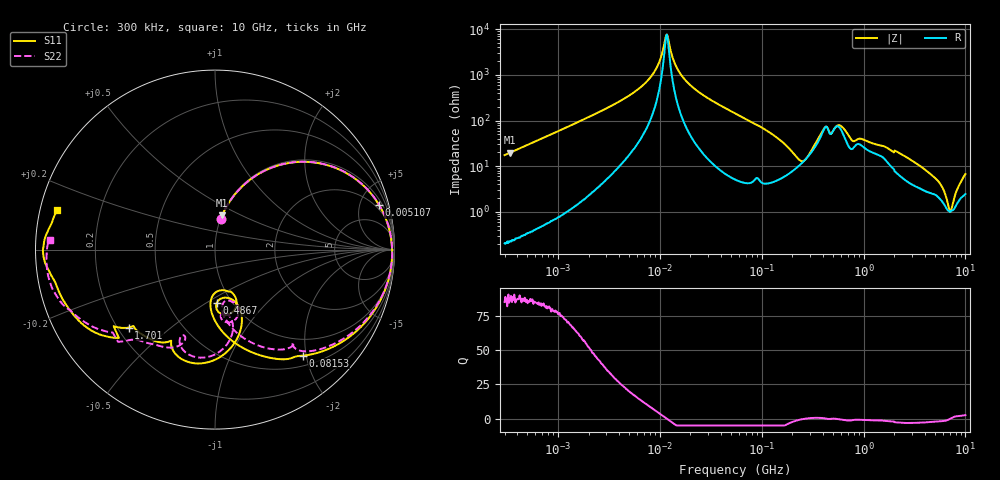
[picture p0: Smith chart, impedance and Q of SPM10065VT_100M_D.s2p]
! S-Parameter Data Generated by TDK Corporation
! Copyright(C) 2020 TDK Corporation.
! All Rights Reserved.
! TDK P/N: SPM10065VT-100M-D (Inductor)
! Property: L=10uH at 100kHz
! Size(LxWxT): 10.5x10x6.5mm
! Model Type: s2p (Touchstone File Format Version 1.0)
! Frequency: DC=Yes Start=0.3MHz Stop=10000MHz 802points Log-sweep
! Model Generated on Apr. 23, 2020
! Port Assignments:
!  1 ---@@@--- 2
! Applicable Conditions:
!  Temperature = 25 degC
!  DC Bias Current = 0 A
!  Small Signal Operation
! Terms and conditions regarding TDK Simulation Models
! (1)This simulation model is being provided solely for informational purposes. Please refer to the specifications of the products in terms of detailed characteristics of such products.
! (2)In no event shall TDK Corporation of any of its subsidiaries be liable for any loss or damage arising, directly or indirectly,
!  From any information contained in this simulation model, including, but not limited to loss or damages arising from any inaccuracies, omissions or errors in connection with such information.
! (3)Any and all copyrights on this simulation model are owned by TDK Corporation.
!  Duplication or redistribution of this simulation model without prior written permission from TDK Corporation is prohibited.
! (4)This simulation model is subject to any modification or change without any prior notice.
! (5)Neither TDK Corporation nor any of its subsidiaries shall make any warranty, express or implied,
!  Including but not limited to the correctness, implied warranties of merchantability and fitness for a particular purpose with respect to this simulation models.
! (6)The use of this simulation model shall be deemed to have consented to the terms and conditions hereof.
# Hz S MA R 50
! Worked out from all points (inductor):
!   801 points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, 300 kHz to 10 GHz, reference 50 ohm
!   read as 1/Y11, port 2 shorted: L = 9.25 uH near 318.3 kHz
!   highest Q = 88.4 at 341.3 kHz (marker M1), where L = 9.27 uH
!   self-resonance near 11.58 MHz
!   S11 on the Smith chart (normalised r, x): 300 kHz: 1.00, +0.35; 5.107 MHz: 1.49, +7.21; 81.53 MHz: 0.68, -1.93; 486.7 MHz: 0.85, -0.56; 1.701 GHz: 0.24, -0.36; 10 GHz: 0.05, +0.12
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300000  0.1728 79.7  0.9824 -9.8  0.9826 -9.9  0.1728 79.6
341258  0.1951 78.3  0.978 -11.2  0.9785 -11.2  0.195 78.2
1713600  0.7024 44.1  0.7001 -44.9  0.6998 -44.9  0.7026 44.2
5106625  0.9475 15.2  0.2767 -72.0  0.2767 -72.0  0.9478 15.3
9671944  0.9834 3.2  0.08616 -78.2  0.08615 -78.2  0.9836 3.6
1.35567e7  0.9872 -2.5  0.01278 11.0  0.01279 11.0  0.9874 -2.0
1.626666e7  0.9859 -5.7  0.05175 70.7  0.05174 70.7  0.9861 -5.1
2.036513e7  0.9808 -9.9  0.1113 74.0  0.1113 74.0  0.9811 -9.1
5.477226e7  0.8766 -35.7  0.4434 52.7  0.4432 52.7  0.8761 -34.0
8.153051e7  0.7665 -50.4  0.5978 36.4  0.5977 36.4  0.745 -49.4
1.765741e8  0.4661 -84.2  0.8088 1.2  0.8086 1.2  0.4753 -75.6
3.126428e8  0.2561 -92.8  0.7956 -33.5  0.7953 -33.5  0.3011 -81.2
3.910695e8  0.2392 -74.1  0.7068 -52.0  0.7066 -52.0  0.3056 -71.9
4.866838e8  0.2976 -88.3  0.5468 -57.3  0.5466 -57.3  0.3879 -84.7
5.99416e8  0.4621 -71.8  0.4513 -69.8  0.4512 -69.8  0.4371 -76.8
7.235338e8  0.6382 -96.8  0.3599 -64.0  0.3598 -64.0  0.6079 -97.9
9.101824e8  0.5643 -115.8  0.4251 -80.9  0.4249 -80.9  0.529 -108.4
1.701119e9  0.6485 -138.0  0.2566 -136.5  0.2564 -136.5  0.686 -132.9
1.767019e9  0.6634 -138.9  0.2415 -141.4  0.2413 -141.4  0.6976 -133.6
2.477118e9  0.8002 -143.9  0.1198 178.7  0.1197 178.7  0.8043 -147.6
5.040844e9  0.909 -168.6  0.01223 166.1  0.01227 166.3  0.9205 -164.0
1e10  0.9072 165.9  0.01842 146.5  0.01843 146.9  0.9193 176.6
